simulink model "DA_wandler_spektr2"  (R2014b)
settings: Solver=ode45  StartTime=0.0  StopTime=3*Tblock  RelTol=1e-3
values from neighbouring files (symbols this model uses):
  ampl1 = 1e-4    (= 0.0001)    [ad_test_2.m]    (also in ad_test_3.m; DA_wandler_spektr_1.m = 1; DA_wandler_spektr_2.m = 1; fourier_reihe1.m = 5)
  ampl2 = 1e-5    (= 1e-05)    [ad_test_2.m]    (also in ad_test_3.m; DA_wandler_spektr_1.m = 1; DA_wandler_spektr_2.m = 1; fourier_reihe1.m = 12)
  f1 = 10    [DA_wandler_spektr_1.m]    (also in DA_wandler_spektr_2.m; fourier_reihe1.m = 100; fourier_reihe2.m = 100; mehrdeutigkeit_1.m = -200)
  f2 = 40    [DA_wandler_spektr_1.m]    (also in DA_wandler_spektr_2.m; fourier_reihe1.m = ',num2str(f2),     ' Hz; fourier_reihe2.m = 200; mehrdeutigkeit_1.m = 1800)
  fs = 4000    [abtast_rate_1.m]    (also in ad_test_12.m = ',     num2str(fs),'; ad_test_2.m = ',     num2str(fs),'; ad_test_3.m = ',     num2str(fs),'; DA_wandler_spektr_1.m = 100)
  N = 4*1024    (= 4096)    [ad_test_12.m]    (also in ad_test_2.m; ad_test_3.m; DA_wandler_spektr_1.m = 1000; DA_wandler_spektr_2.m = 1024)
  nfft = 2^p2    [DA_wandler_spektr_1.m]    (also in DA_wandler_spektr_2.m; PSD_korrelation_1.m = 2^(nextpow2(2*lag_max)); welch_1.m = 256; zero_padd1.m = ',num2str(nfft),')
  Ts = 1/fs    (= 0.00025)    [abtast_rate_1.m]    (also in ad_test_12.m = 0.0009765625; ad_test_2.m = 0.00048828125; ad_test_3.m = 0.00048828125; DA_wandler_spektr_1.m = 0.01)
undefined symbols (not defined in the file or in its folder): get
libraries: dspspect3 x2, dspsnks4 x2

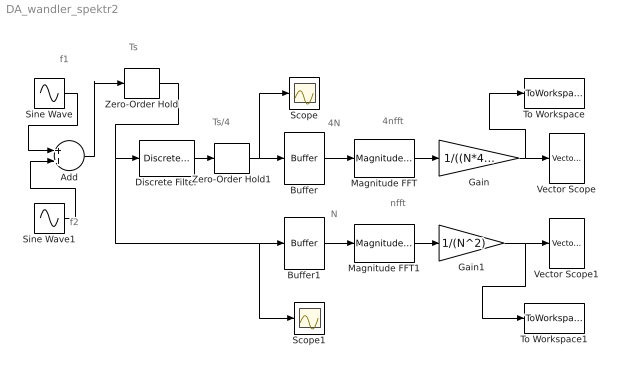
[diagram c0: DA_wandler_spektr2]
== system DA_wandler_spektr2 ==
  note: nfft
  note: 4nfft
  note: N
  note: 4N
  note: f2
  note: f1
  note: Ts/4
  note: Ts
  Add : Sum
  Buffer : Buffer  N=4*N  TreatMby1Signals=One channel
  Buffer1 : Buffer  N=N  TreatMby1Signals=One channel
  Discrete Filter : DiscreteFilter  Numerator=[-1, 18, -1]/16  Denominator=[1]
  Gain : Gain  Gain=1/((N*4)^2)
  Gain1 : Gain  Gain=1/(N^2)
  Magnitude FFT : dspspect3/Magnitude FFT  mag_or_magsq=Magnitude squared  FFTImplementation=Auto  fftLenInherit=off  fftsize=4*nfft  WrapInput=on
  Magnitude FFT1 : dspspect3/Magnitude FFT  mag_or_magsq=Magnitude squared  FFTImplementation=Auto  fftLenInherit=off  fftsize=nfft  WrapInput=on
  Scope : Scope
  Scope1 : Scope
  Sine Wave : Sin  Amplitude=ampl1  Frequency=2*pi*f1  SampleTime=0
  Sine Wave1 : Sin  Amplitude=ampl2  Frequency=2*pi*f2  SampleTime=0
  To Workspace : ToWorkspace  VariableName=Y  SaveFormat=Structure  SampleTime=-1
  To Workspace1 : ToWorkspace  VariableName=Y1  SaveFormat=Structure  SampleTime=-1
  Vector Scope : dspsnks4/Vector Scope  ScopeProperties=on  Domain=Frequency  HorizSpan=1  DisplayProperties=off  AxisGrid=on  Memory=off  FrameNumber=on  AxisLegend=off  AxisZoom=off  OpenScopeAtSimStart=on  OpenScopeImmediately=off  FigPos=get(0,'defaultfigureposition')  AxisProperties=off  XUnits=Hertz  XRange=[0...Fs]  InheritXIncr=off  XIncr=Ts/4  XLabel=Time  XLimit=User-defined  XMin=0  XMax=fs*4  XStart=0  YUnits=dB  YLabel=Amplitude  LineProperties=off  XAxisParamsVer=6.9
  Vector Scope1 : dspsnks4/Vector Scope  ScopeProperties=on  Domain=Frequency  HorizSpan=1  DisplayProperties=off  AxisGrid=on  Memory=off  FrameNumber=on  AxisLegend=off  AxisZoom=off  OpenScopeAtSimStart=on  OpenScopeImmediately=off  FigPos=[167 289 560 420]  AxisProperties=off  XUnits=Hertz  XRange=[0...Fs]  InheritXIncr=off  XIncr=Ts  XLabel=Time  XLimit=User-defined  XMin=0  XMax=fs  XStart=0  YUnits=dB  YLabel=Amplitude  LineProperties=off  XAxisParamsVer=6.9
  Zero-Order Hold : ZeroOrderHold  SampleTime=Ts
  Zero-Order Hold1 : ZeroOrderHold  SampleTime=Ts/4
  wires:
  Buffer/1 -> Magnitude FFT/1
  Magnitude FFT/1 -> Gain/1
  Gain/1 -> To Workspace/1, Vector Scope/1
  Zero-Order Hold1/1 -> Scope/1, Buffer/1
  Buffer1/1 -> Magnitude FFT1/1
  Magnitude FFT1/1 -> Gain1/1
  Gain1/1 -> To Workspace1/1, Vector Scope1/1
  Zero-Order Hold/1 -> Scope1/1, Buffer1/1, Discrete Filter/1
  Add/1 -> Zero-Order Hold/1
  Sine Wave/1 -> Add/1
  Sine Wave1/1 -> Add/2
  Discrete Filter/1 -> Zero-Order Hold1/1
